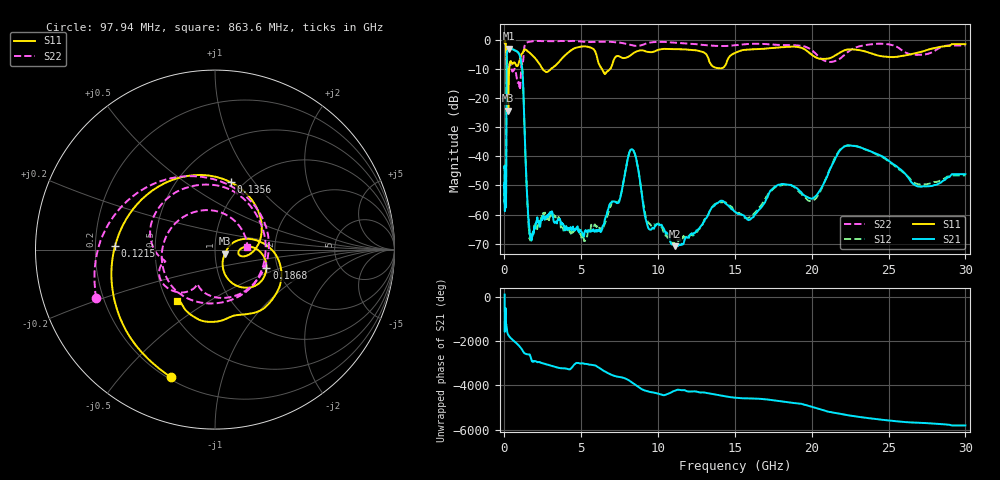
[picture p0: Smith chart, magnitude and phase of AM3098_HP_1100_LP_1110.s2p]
! Date/Time: Thu, Feb 28, 2019 8:44 AM
! Network Analyzer: Agilent Technologies E8364B Rev: A.07.50.67
! Sweep from 0.010 to 30.000 GHz, 1601 Points, Sweep Type: LOG
! Power Supply: 5.023 V, 0.002 A
# Hz S DB R 50
!freq MagS11 AngS11 MagS21 AngS21 MagS12 AngS12 MagS22 AngS22
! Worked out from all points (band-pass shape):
!   1601 points, 10 MHz to 30 GHz, reference 50 ohm
!   highest |S21| = -3.12 dB at 265.1 MHz (marker M1); lowest = -70.8 dB at 11.08 GHz (marker M2)
!   |S21| within 3 dB of the highest: 149.1 MHz to 1.027 GHz (877.9 MHz wide, 149 % of centre)
!   lowest |S11| = -24.4 dB at 248.4 MHz (marker M3), VSWR 1.13, Z = 55.9 - j2.49 ohm
!   |S11| at or under -10 dB: 140.1 MHz to 310.4 MHz (170.2 MHz wide, 75.6 % of centre); 2.472 GHz to 3.04 GHz (568.5 MHz wide, 20.6 % of centre); 6.334 GHz to 6.895 GHz (561.1 MHz wide, 8.48 % of centre)
!   |S22| runs from -17.2 to -0.5 dB; largest |S21 - S12| = 0.013
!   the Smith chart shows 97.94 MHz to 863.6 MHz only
!   S11 on the Smith chart (normalised r, x): 97.94 MHz: 0.21, -0.69; 121.5 MHz: 0.28, +0.02; 135.6 MHz: 0.87, +0.77; 186.8 MHz: 1.74, -0.40; 863.6 MHz: 0.57, -0.37
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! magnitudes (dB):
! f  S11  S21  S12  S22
! 10 MHz  -0.4  -44.1  -44.3  -0.6
! 38.04 MHz  -0.4  -56.8  -55.9  -0.9
! 97.94 MHz  -2.5  -54.8  -51.7  -2.9
! 121.5 MHz  -5.1  -35.0  -34.8  -6.6
! 135.6 MHz  -8.3  -14.0  -13.9  -10.6
! 144.7 MHz  -12.2  -7.5  -7.4  -11.7
! 186.8 MHz  -10.3  -3.9  -3.8  -9.5
! 248.4 MHz  -24.4  -3.1  -3.1  -10.9
! 265.1 MHz  -18.6  -3.1  -3.1  -10.7
! 550.5 MHz  -8.2  -3.4  -3.4  -10.9
! 863.6 MHz  -9.0  -4.3  -4.2  -14.8
! 1.178 GHz  -4.7  -11.3  -11.2  -8.7
! 1.622 GHz  -4.5  -64.6  -67.7  -0.8
! 2.084 GHz  -6.9  -62.2  -63.8  -0.5
! 6.11 GHz  -7.9  -65.2  -64.2  -0.8
! 7.926 GHz  -6.2  -43.5  -43.7  -1.5
! 8.416 GHz  -4.6  -38.3  -38.2  -2.1
! 9.396 GHz  -4.3  -64.9  -62.9  -1.1
! 11.08 GHz  -3.3  -70.8  -70.0  -1.1
! 20 GHz  -5.3  -54.6  -55.4  -3.6
! 22.56 GHz  -3.4  -36.3  -36.3  -3.5
! 30 GHz  -1.6  -46.2  -46.6  -2.0
